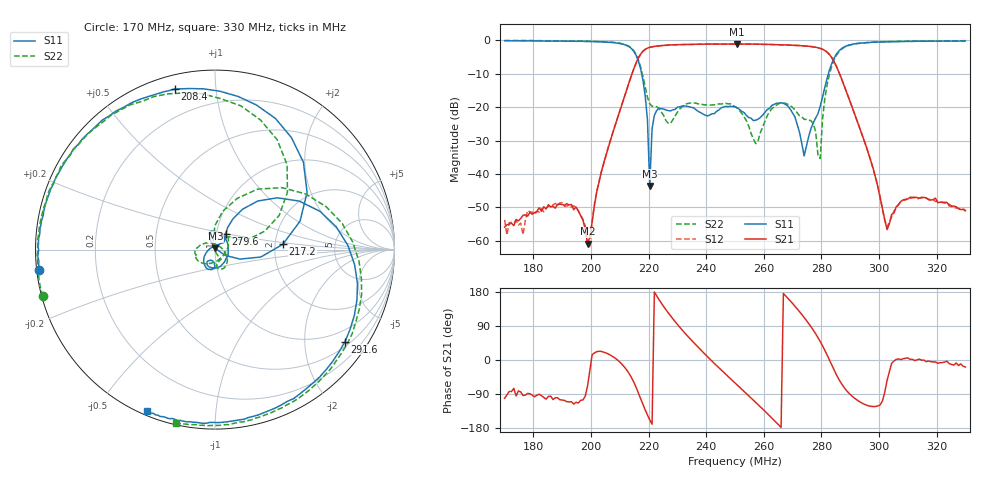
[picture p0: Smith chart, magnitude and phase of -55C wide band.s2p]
!Agilent Technologies,E8362C,SG49020144,A.09.33.09
!Agilent E8362C: A.09.33.09
!Date: Friday, October 10, 2025 10:25:34
!Correction: S11(Full 2 Port(1,2))
!S21(Full 2 Port(1,2))
!S12(Full 2 Port(1,2))
!S22(Full 2 Port(1,2))
!S2P File: Measurements: S11, S21, S12, S22:
# Hz S  dB  R 50
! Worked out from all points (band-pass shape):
!   201 points, 170 MHz to 330 MHz, reference 50 ohm
!   highest |S21| = -1.09 dB at 250.8 MHz (marker M1); lowest = -60.9 dB at 198.8 MHz (marker M2)
!   |S21| within 3 dB of the highest: 217.3 MHz to 282.6 MHz (65.35 MHz wide, 26.1 % of centre)
!   lowest |S11| = -43.6 dB at 220.4 MHz (marker M3), VSWR 1.01, Z = 50.2 + j0.633 ohm
!   |S11| at or under -10 dB: 217.6 MHz to 282.4 MHz (64.85 MHz wide, 25.9 % of centre)
!   |S22| runs from -35.4 to 0.0 dB; largest |S21 - S12| = 0.0077
!   S11 on the Smith chart (normalised r, x): 170 MHz: 0.01, -0.06; 208.4 MHz: 0.07, +0.78; 217.2 MHz: 2.21, +0.15; 279.6 MHz: 1.11, +0.19; 291.6 MHz: 0.63, -3.03; 330 MHz: 0.02, -0.67
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1.7e8  -0.11 -173.5  -55.94 -101.2  -53.78 -81.8  -0.05 -164.9
1.972e8  -0.28 144.5  -53.81 -105.4  -53.66 -104.2  -0.23 155.6
1.988e8  -0.33 140.4  -60.87 -68.7  -61.36 -74.5  -0.21 151.7
2.084e8  -0.71 104.0  -25.39 4.9  -25.39 4.5  -0.72 116.0
2.172e8  -8.42 4.5  -4.19 -101.3  -4.17 -101.3  -7.85 28.0
2.196e8  -23.77 -29.7  -2.33 -145.1  -2.35 -145.2  -17.05 23.4
2.204e8  -43.59 72.4  -2.06 -158.0  -2.12 -158.1  -19.00 36.4
2.212e8  -26.52 117.5  -1.96 -169.6  -1.92 -169.5  -19.73 46.0
2.236e8  -20.33 104.8  -1.65 159.5  -1.66 159.7  -20.39 38.4
2.3e8  -20.00 109.7  -1.29 93.8  -1.32 94.0  -21.53 -112.0
2.38e8  -21.61 43.0  -1.12 27.3  -1.18 27.2  -18.98 -162.6
2.5e8  -19.87 -110.3  -1.11 -60.4  -1.13 -60.4  -19.82 175.1
2.508e8  -20.18 -115.1  -1.09 -66.1  -1.12 -66.2  -20.33 172.5
2.572e8  -23.92 -106.6  -1.16 -111.9  -1.16 -112.0  -30.93 63.6
2.66e8  -18.70 -109.3  -1.34 -178.0  -1.34 -178.1  -18.74 -66.0
2.74e8  -34.62 119.6  -1.70 112.4  -1.68 112.4  -23.65 -67.7
2.772e8  -24.70 39.6  -1.95 78.5  -1.97 78.5  -25.06 -60.5
2.796e8  -19.72 55.5  -2.41 48.7  -2.43 48.7  -35.40 110.2
2.836e8  -6.91 39.8  -5.19 -13.4  -5.20 -13.6  -7.70 54.8
2.916e8  -1.04 -35.3  -22.17 -101.4  -22.23 -101.6  -1.09 -27.3
3.036e8  -0.42 -76.9  -54.96 -31.0  -54.46 -33.2  -0.38 -68.9
3.3e8  -0.21 -112.7  -51.07 -18.5  -50.82 -15.6  -0.10 -102.8
